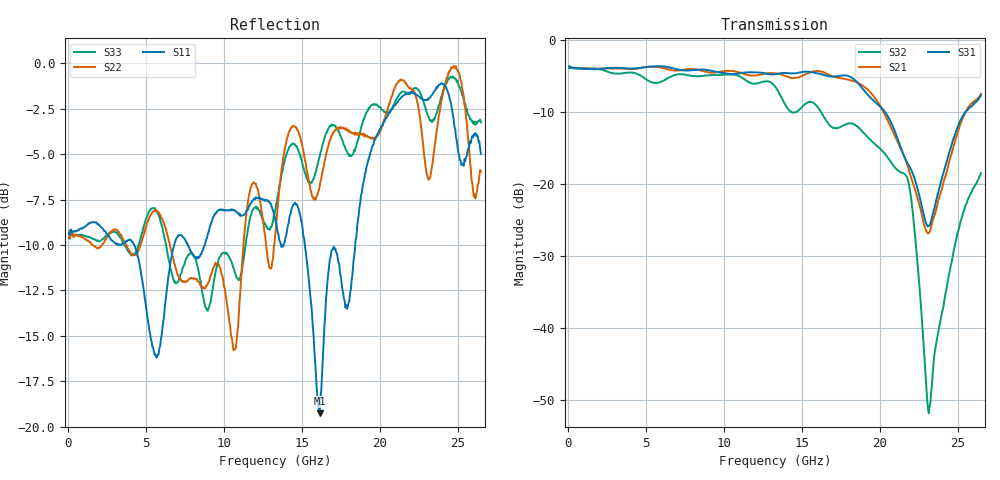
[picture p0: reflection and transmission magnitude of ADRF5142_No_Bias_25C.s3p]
! Device: ADRF5142
! Description: Silicon, SPDT Switch, Reflective
! Frequency: 8.00 GHz - 11.00 GHz
! Ports:
!  RFC = Port 1
!  RF1 = Port 2
!  RF2 = Port 3
! VDD = 0V
! VSS = 0V
! Temp = 25C
! Data:  Data was collected using an calibrated 4 port network analyzer.
!  The reference plane is the package pins of ADRF5142 switch.
! Notes: Analog Devices supplies this data as a sample of measured data
!  for this product.  Your particular data for this product may vary.
!  Data was taken at 25 degrees C.
!  Analog Devices reserves the right to change this data at anytime.
# HZ S DB R 50
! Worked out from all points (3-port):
!   530 points, 50 MHz to 26.5 GHz, reference 50 ohm
!   strongest paths, dB at 50 MHz, 6.65 GHz, 13.3 GHz, 19.9 GHz, 26.5 GHz:
!     S31: -3.7, -3.9, -4.8, -9.0, -7.7
!     S21: -3.8, -4.2, -4.7, -8.7, -7.5
!     S32: -4.0, -5.1, -6.6, -14.8, -18.5
!   lowest |S11| = -19.3 dB at 16.15 GHz (marker M1), VSWR 1.24, Z = 40.4 - j1.99 ohm
!   |S11| at or under -10 dB: 4.233 GHz to 6.802 GHz (2.569 GHz wide, 46.6 % of centre); 7.683 GHz to 8.759 GHz (1.076 GHz wide, 13.1 % of centre); 15.19 GHz to 18.43 GHz (3.236 GHz wide, 19.3 % of centre)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
5e7  -9.37 175.7  -3.77 -2.3  -3.67 -3.8
     -3.77 -2.3  -9.24 175.2  -3.96 -4.9
     -3.67 -3.8  -3.96 -4.9  -9.64 174.1
3.4e9  -10.00 44.3  -4.00 -178.8  -3.92 -177.4
       -4.00 -178.8  -9.44 -65.4  -4.69 123.2
       -3.92 -177.4  -4.69 123.2  -9.63 -62.3
6.65e9  -10.58 -68.2  -4.24 7.6  -3.92 9.0
        -4.24 7.6  -10.48 92.6  -5.05 -95.4
        -3.92 9.0  -5.05 -95.4  -11.60 96.2
1.02e10  -8.10 160.5  -4.32 -179.3  -4.71 -176.5
         -4.32 -179.3  -13.28 174.2  -4.84 9.7
         -4.71 -176.5  -4.84 9.7  -10.49 176.7
1.33e10  -8.64 34.6  -4.66 15.2  -4.79 21.5
         -4.66 15.2  -9.35 -108.7  -6.55 135.6
         -4.79 21.5  -6.55 135.6  -8.05 -86.5
1.615e10  -19.26 -167.1  -4.37 -142.3  -4.74 -137.3
          -4.37 -142.3  -6.74 91.0  -9.74 -62.0
          -4.74 -137.3  -9.74 -62.0  -5.11 101.1
2.01e10  -3.50 -152.0  -9.45 -25.7  -9.41 -11.6
         -9.45 -25.7  -3.60 -123.1  -15.29 17.6
         -9.41 -11.6  -15.29 17.6  -2.54 -87.2
2.315e10  -1.93 17.8  -26.85 -114.2  -25.89 -105.8
          -26.85 -114.2  -6.41 83.9  -51.86 -150.7
          -25.89 -105.8  -51.86 -150.7  -2.98 117.6
2.5e10  -4.57 -89.2  -12.95 -145.1  -12.13 -142.6
        -12.95 -145.1  -0.36 21.1  -26.87 -137.4
        -12.13 -142.6  -26.87 -137.4  -0.98 24.2
2.65e10  -4.99 150.0  -7.53 109.0  -7.71 124.3
         -7.53 109.0  -5.96 -103.5  -18.52 106.5
         -7.71 124.3  -18.52 106.5  -3.25 -61.3
